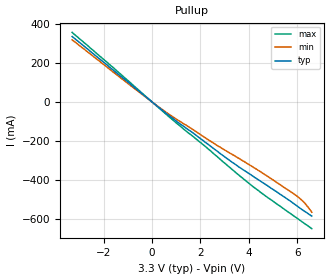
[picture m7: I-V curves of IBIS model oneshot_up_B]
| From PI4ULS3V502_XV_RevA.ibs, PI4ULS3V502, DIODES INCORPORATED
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[Model]   oneshot_up_B
Model_type  Open_source
Vref = 0
Rref = 50
Vmeas = 1.65
C_comp   8.864pF   8.757pF   8.982pF
[Voltage Range]   3.30V   3.0V   3.6V
[Temperature Range]   25   85   -40
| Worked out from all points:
|   slope of the pullup table from 0 to 0.495 V, typ, clamps not added: 10 ohm
[Pullup]
-3.3V     334mA      317mA      355mA
0V        450pA      8.5nA      90.7pA
1.1V      -107mA     -95.3mA    -117mA
2.2V      -206mA     -183mA     -227mA
3.3V      -307mA     -267mA     -344mA
4.2V      -382mA     -335mA     -435mA
5.8V      -514mA     -464mA     -577mA
6.3V      -558mA     -515mA     -621mA
6.6V      -583mA     -563mA     -647mA
[Ramp]
| variable   typ   min   max
dV/dt_r   1.63/172.9E-12   1.46/211.9E-12   1.81/143.9E-12
dV/dt_f   1.63/587.8E-12   1.46/567.0E-12   1.81/577.0E-12
R_load = 50
